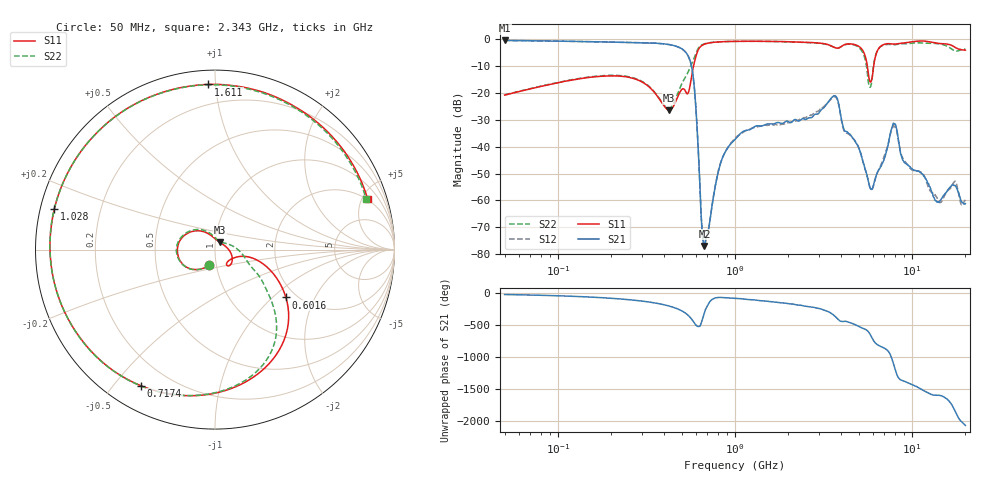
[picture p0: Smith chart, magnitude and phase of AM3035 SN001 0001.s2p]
# Hz S DB R 50
!freq MagS11 AngS11 MagS21 AngS21 MagS12 AngS12 MagS22 AngS22
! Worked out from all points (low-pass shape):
!   1601 points, 50 MHz to 20.05 GHz, reference 50 ohm
!   highest |S21| = -0.36 dB at 50 MHz (marker M1); lowest = -77.0 dB at 673.1 MHz (marker M2)
!   |S21| within 3 dB of the highest: start of sweep to 497.8 MHz
!   lowest |S11| = -26.3 dB at 426.2 MHz (marker M3), VSWR 1.10, Z = 52.5 + j4.24 ohm
!   |S11| at or under -10 dB: start of sweep to 583.3 MHz; 5.602 GHz to 6.078 GHz (476.9 MHz wide, 8.17 % of centre)
!   |S22| runs from -25.8 to -0.7 dB; largest |S21 - S12| = 0.0061
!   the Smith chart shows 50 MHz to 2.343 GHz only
!   S11 on the Smith chart (normalised r, x): 50 MHz: 0.92, -0.16; 601.6 MHz: 1.77, -1.22; 717.4 MHz: 0.10, -0.59; 1.028 GHz: 0.04, +0.12; 1.611 GHz: 0.08, +0.96; 2.343 GHz: 1.96, +5.57
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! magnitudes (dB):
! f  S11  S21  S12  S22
! 50 MHz  -20.7  -0.4  -0.4  -20.6
! 135.9 MHz  -14.5  -0.8  -0.8  -14.4
! 369.6 MHz  -21.7  -1.4  -1.5  -21.5
! 426.2 MHz  -26.3  -1.9  -1.9  -25.7
! 549.8 MHz  -19.1  -6.7  -6.8  -11.5
! 601.6 MHz  -6.4  -25.2  -25.1  -5.3
! 650.8 MHz  -2.3  -70.1  -70.0  -2.0
! 673.1 MHz  -1.8  -77.0  -77.0  -1.6
! 717.4 MHz  -1.3  -68.8  -69.2  -1.2
! 824 MHz  -0.9  -46.8  -46.6  -0.9
! 1.005 GHz  -0.7  -37.2  -36.7  -0.7
! 1.028 GHz  -0.7  -36.5  -36.1  -0.7
! 1.611 GHz  -0.7  -31.5  -31.7  -0.7
! 2.343 GHz  -1.0  -30.1  -29.7  -1.0
! 2.722 GHz  -1.1  -29.0  -28.2  -1.2
! 3.715 GHz  -3.1  -21.1  -21.5  -3.2
! 5.032 GHz  -2.7  -40.8  -40.6  -3.1
! 5.89 GHz  -15.6  -55.9  -56.0  -16.8
! 7.402 GHz  -1.6  -37.9  -38.0  -1.8
! 8.008 GHz  -1.7  -31.5  -32.5  -1.9
! 13.79 GHz  -1.3  -60.3  -58.8  -1.5
! 20.05 GHz  -3.9  -61.2  -59.8  -3.6
